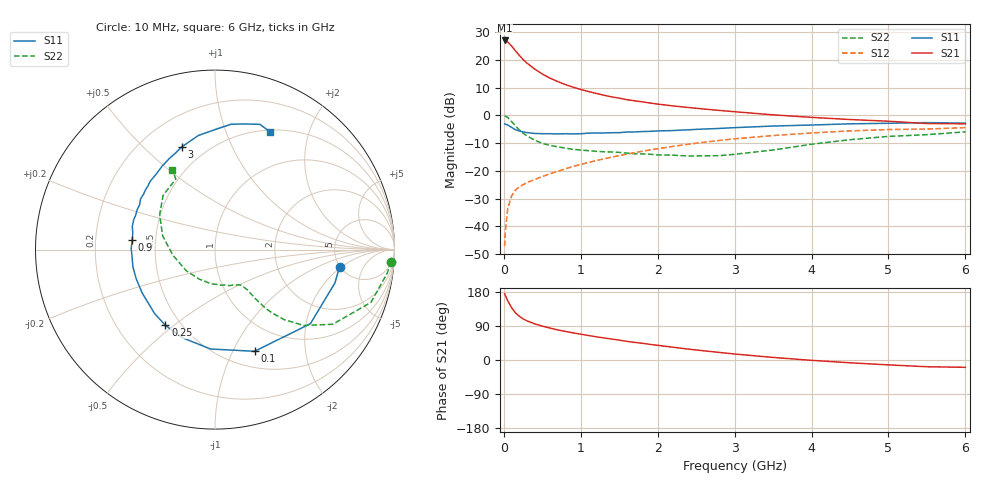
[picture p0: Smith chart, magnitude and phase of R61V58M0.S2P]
! SIEMENS Small Signal Semiconductors
! BFR193
! Si NPN RF Bipolar Junction Transistor in SOT23
! VCE = 1.5 V  IC = 8 mA
! Common Emitter S-Parameters:  May  1996
# GHz  S  MA  R  50
!  f  S11  S21  S12  S22
! GHz  MAG  ANG  MAG  ANG  MAG  ANG  MAG  ANG
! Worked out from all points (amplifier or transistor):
!   36 points, 10 MHz to 6 GHz, reference 50 ohm
!   highest |S21| = 27.0 dB at 10 MHz (marker M1)
!   |S21| within 3 dB of that: start of sweep to 129.2 MHz
!   unconditionally stable (mu >= 1): 763.2 MHz to 2.03 GHz
!   at 250 MHz: K = 0.58, MSG = 22.6 dB, |S12| = -25.0 dB
!   at 1.4 GHz: K = 1.05, MAG = 9.5 dB, |S12| = -15.1 dB
!   at 6 GHz: K = 0.96, MSG = 0.7 dB, |S12| = -4.4 dB
!   S11 on the Smith chart (normalised r, x): 10 MHz: 4.96, -1.85; 100 MHz: 0.68, -1.22; 250 MHz: 0.41, -0.47; 900 MHz: 0.37, +0.05; 3 GHz: 0.37, +0.66; 6 GHz: 0.52, +1.44
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0.01  0.7006 -7.8  22.39 175.4  0.0044 86.6  0.9837 -3.9
0.02  0.6937 -15.5  22.06 170.2  0.0083 80.2  0.969 -7.7
0.05  0.6731 -37.8  21.15 156.6  0.0206 72.7  0.9173 -18.7
0.1  0.6082 -68.7  17.84 138.3  0.0353 61.6  0.7766 -32.4
0.15  0.5543 -92.5  14.58 124.7  0.045 55.4  0.6508 -40.5
0.2  0.5237 -110.1  12.15 115.4  0.0512 52.4  0.5498 -45.3
0.25  0.5044 -123.2  10.18 108.6  0.0564 51.4  0.4769 -47.9
0.3  0.4902 -133.3  8.764 103.4  0.0614 51.5  0.4277 -49.3
0.4  0.4723 -149.2  6.85 95.6  0.0699 53.1  0.357 -50.5
0.5  0.4683 -159.5  5.561 89.3  0.0791 54.9  0.3129 -50.9
0.6  0.4674 -168.0  4.69 84.2  0.0886 56.0  0.2884 -51.2
0.7  0.4638 -174.8  4.076 79.4  0.0983 57.5  0.2715 -52.0
0.9  0.4643 173.3  3.224 71.6  0.1202 59.2  0.2443 -54.1
1.1  0.4786 164.3  2.692 64.6  0.1418 59.9  0.2314 -58.2
1.3  0.4822 156.2  2.308 58.2  0.165 59.5  0.2211 -62.6
1.6  0.5017 145.8  1.919 49.2  0.2002 58.1  0.2093 -71.9
2.2  0.533 128.0  1.481 33.7  0.2765 52.8  0.192 -96.5
3  0.6013 108.0  1.164 15.8  0.3782 42.1  0.1991 -143.7
3.5  0.6425 98.3  1.023 6.8  0.433 34.3  0.2378 -172.9
4.5  0.7048 82.6  0.842 -7.4  0.5253 18.9  0.3648 147.7
5.5  0.7415 70.3  0.713 -17.8  0.5668 3.3  0.4494 119.1
6  0.7244 64.9  0.705 -19.3  0.6026 -1.2  0.5051 118.0
